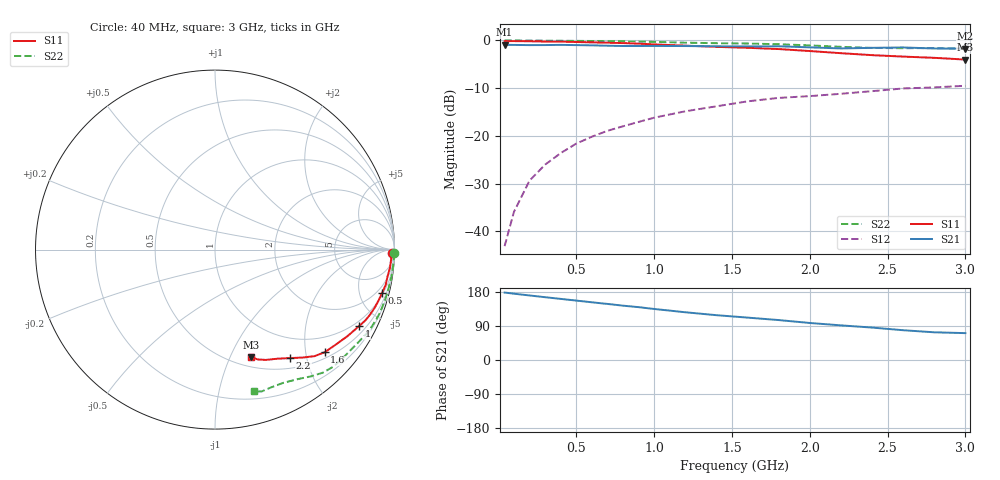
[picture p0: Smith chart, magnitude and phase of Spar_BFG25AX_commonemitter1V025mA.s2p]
! Filename:  BFG25AXB.S2P  Version:  2.0
! NXP part #: BFG25A/X  Date: May 1990
! Bias condition: Vce=1V, Ic=0.25mA
#  MHz  S  MA  R  50
! Freq  S11  S21  S12  S22  !GUM [dB]
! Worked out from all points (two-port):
!   21 points, 40 MHz to 3 GHz, reference 50 ohm
!   highest |S21| = -0.92 dB at 40 MHz (marker M1); lowest = -1.7 dB at 3 GHz (marker M2)
!   |S21| within 3 dB of the highest: start of sweep to end of sweep
!   lowest |S11| = -4.0 dB at 3 GHz (marker M3), VSWR 4.41, Z = 30.2 - j59.8 ohm
!   |S11| at or under -10 dB: nowhere
!   |S22| runs from -1.7 to 0.0 dB; largest |S21 - S12| = 0.9
!   S11 on the Smith chart (normalised r, x): 40 MHz: 46, -60; 500 MHz: 1.19, -7.68; 1 GHz: 0.79, -3.84; 1.6 GHz: 0.63, -2.39; 2.2 GHz: 0.65, -1.72; 3 GHz: 0.60, -1.20
40  0.984 -1.2  0.9 178.0  0.007 85.2  0.999 -1.2
100  0.983 -3.0  0.897 175.0  0.016 88.0  0.998 -3.1
200  0.98 -5.9  0.893 170.3  0.034 85.0  0.996 -6.1
300  0.973 -8.8  0.894 165.7  0.05 82.7  0.994 -9.1
400  0.971 -11.7  0.898 161.3  0.066 80.4  0.991 -12.2
500  0.962 -14.5  0.893 156.8  0.083 78.7  0.989 -15.2
600  0.954 -17.4  0.888 152.3  0.098 76.9  0.986 -18.1
700  0.947 -20.0  0.88 148.0  0.113 75.0  0.984 -20.9
800  0.937 -22.7  0.874 143.4  0.126 73.2  0.979 -23.5
900  0.926 -25.2  0.874 139.5  0.14 71.1  0.973 -26.2
1000  0.908 -28.1  0.875 134.7  0.155 69.2  0.966 -28.9
1200  0.882 -33.1  0.873 126.0  0.181 64.3  0.947 -34.2
1400  0.856 -38.2  0.868 118.3  0.204 60.8  0.935 -39.5
1600  0.837 -43.1  0.866 111.9  0.23 58.2  0.928 -44.5
1800  0.812 -47.0  0.868 105.4  0.25 54.4  0.912 -48.7
2000  0.774 -51.0  0.846 97.7  0.261 50.9  0.887 -52.7
2200  0.735 -55.3  0.824 91.4  0.276 48.0  0.857 -57.3
2400  0.701 -60.1  0.836 85.6  0.294 43.8  0.834 -62.9
2600  0.677 -65.2  0.844 78.6  0.314 40.0  0.829 -68.0
2800  0.657 -68.7  0.823 73.1  0.322 37.9  0.832 -71.8
3000  0.63 -71.6  0.821 70.9  0.335 37.7  0.819 -74.8
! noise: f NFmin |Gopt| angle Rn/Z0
500  1.4  0.92  4  4
1000  1.6  0.81  13  3.8
2000  1.7  0.8  39  2.4
